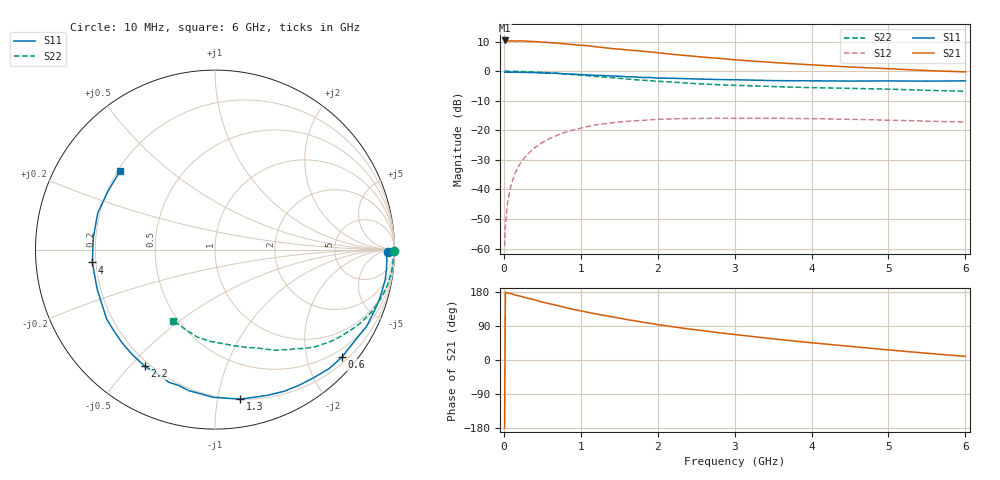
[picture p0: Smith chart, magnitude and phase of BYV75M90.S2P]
! SIEMENS Small Signal Semiconductors
! BFY420
! Si NPN RF SIEGET Grounded Emitter Transistor in MICRO-X
! VCE = 0.75 V  IC = 0.9 mA
! Common Emitter S-Parameters:  October  1996
# GHz  S  MA  R  50
!  f  S11  S21  S12  S22
! GHz  MAG  ANG  MAG  ANG  MAG  ANG  MAG  ANG
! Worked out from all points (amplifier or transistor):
!   36 points, 10 MHz to 6 GHz, reference 50 ohm
!   highest |S21| = 10.4 dB at 10 MHz (marker M1)
!   |S21| within 3 dB of that: start of sweep to 1.53 GHz
!   unconditionally stable (mu >= 1): 4.592 GHz to end of sweep
!   at 250 MHz: K = 0.03, MSG = 20.0 dB, |S12| = -29.9 dB
!   at 1.4 GHz: K = 0.23, MSG = 12.6 dB, |S12| = -17.5 dB
!   at 6 GHz: K = 1.34, MAG = 5.0 dB, |S12| = -17.2 dB
!   S11 on the Smith chart (normalised r, x): 10 MHz: 45, -16; 600 MHz: 0.32, -2.70; 1.3 GHz: 0.20, -1.16; 2.2 GHz: 0.18, -0.55; 4 GHz: 0.19, -0.05; 6 GHz: 0.21, +0.35
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0.01  0.9616 -0.8  3.309 -179.3  0.0011 93.8  0.9976 -0.4
0.02  0.9547 -1.6  3.274 178.8  0.0024 86.9  0.9999 -0.7
0.05  0.9597 -3.5  3.245 176.8  0.0063 90.1  0.9979 -1.9
0.1  0.9615 -6.8  3.255 175.1  0.0127 85.6  0.9941 -3.8
0.15  0.9631 -10.0  3.229 171.2  0.0194 83.1  0.9928 -5.7
0.25  0.9573 -17.0  3.246 166.3  0.0321 79.4  0.9856 -9.4
0.3  0.9527 -20.0  3.209 163.5  0.0386 77.2  0.9822 -11.3
0.4  0.9468 -26.8  3.166 158.9  0.0506 73.0  0.9702 -14.9
0.5  0.9294 -33.5  3.101 152.7  0.062 68.7  0.9545 -18.4
0.6  0.9269 -40.2  3.04 148.3  0.0732 64.4  0.9378 -21.9
0.9  0.8892 -58.3  2.814 133.7  0.1016 52.7  0.8762 -31.0
1.1  0.8628 -70.2  2.69 125.6  0.1165 45.8  0.8355 -36.8
1.3  0.8446 -80.5  2.507 117.8  0.1289 39.6  0.7943 -41.7
1.6  0.8072 -95.8  2.291 106.6  0.1423 31.2  0.7378 -48.3
1.8  0.7835 -104.9  2.174 99.8  0.1476 26.5  0.704 -51.9
2.2  0.759 -121.1  1.922 87.7  0.1565 17.8  0.6541 -59.1
2.8  0.7222 -141.5  1.647 71.9  0.1601 8.0  0.5884 -68.3
3.5  0.6928 -161.3  1.403 55.8  0.1608 -0.4  0.5502 -77.6
4  0.687 -174.0  1.28 45.5  0.1572 -5.4  0.5266 -84.9
4.5  0.6812 174.1  1.177 36.0  0.1536 -9.8  0.513 -92.4
5.5  0.6792 151.1  1.025 17.8  0.1433 -15.1  0.4747 -110.2
6  0.6866 140.5  0.973 9.5  0.1378 -15.9  0.458 -120.4
